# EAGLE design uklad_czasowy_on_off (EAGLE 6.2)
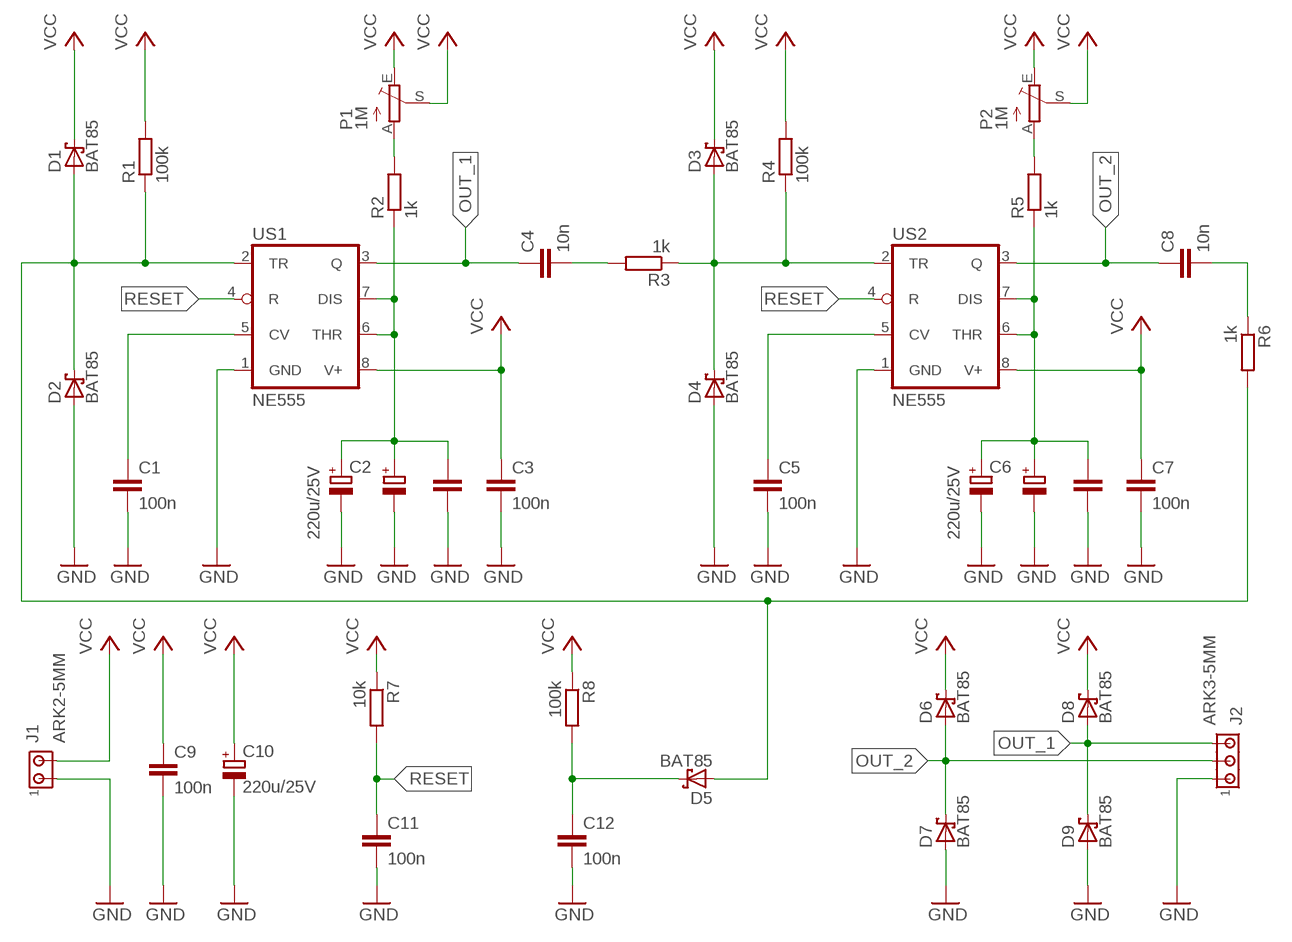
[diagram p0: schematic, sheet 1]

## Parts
C1  100n  C-EU050-025X075  [C050-025X075]
C2  220u/25V  CPOL-EUE3.5-10  [E3,5-10]
C2A  CPOL-EUE2.5-7  [E2,5-7]
C2B  C-EU050-025X075  [C050-025X075]
C3  100n  C-EU050-025X075  [C050-025X075]
C4  10n  C-EU050-025X075  [C050-025X075]
C5  100n  C-EU050-025X075  [C050-025X075]
C6  220u/25V  CPOL-EUE3.5-10  [E3,5-10]
C6A  CPOL-EUE2.5-7  [E2,5-7]
C6B  C-EU050-025X075  [C050-025X075]
C7  100n  C-EU050-025X075  [C050-025X075]
C8  10n  C-EU050-025X075  [C050-025X075]
C9  100n  C-EU050-025X075  [C050-025X075]
C10  220u/25V  CPOL-EUE2.5-6  [E2,5-6]
C11  100n  C-EU050-025X075  [C050-025X075]
C12  100n  C-EU050-025X075  [C050-025X075]
D1  BAT85  SCHOTTKY-DIODEDO35-7  [DO35-7]
D2  BAT85  SCHOTTKY-DIODEDO35-7  [DO35-7]
D3  BAT85  SCHOTTKY-DIODEDO35-7  [DO35-7]
D4  BAT85  SCHOTTKY-DIODEDO35-7  [DO35-7]
D5  BAT85  SCHOTTKY-DIODEDO35-7  [DO35-7]
D6  BAT85  SCHOTTKY-DIODEDO35-7  [DO35-7]
D7  BAT85  SCHOTTKY-DIODEDO35-7  [DO35-7]
D8  BAT85  SCHOTTKY-DIODEDO35-7  [DO35-7]
D9  BAT85  SCHOTTKY-DIODEDO35-7  [DO35-7]
J1  ARK2-5MM  [2PIN-5MM]
J2  ARK3-5MM  [3PIN-5MM]
P1  1M  TRIM_EU-B90P  [SP19L]
P2  1M  TRIM_EU-B90P  [SP19L]
R1  100k  R-EU_0207/7  [0207/7]
R2  1k  R-EU_0207/7  [0207/7]
R3  1k  R-EU_0207/7  [0207/7]
R4  100k  R-EU_0207/7  [0207/7]
R5  1k  R-EU_0207/7  [0207/7]
R6  1k  R-EU_0207/7  [0207/7]
R7  10k  R-EU_0207/7  [0207/7]
R8  100k  R-EU_0207/7  [0207/7]
US1  NE555  LM555N  [DIL08]
US2  NE555  LM555N  [DIL08]

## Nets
GND: C1.2 C2.- C2A.- C2B.2 C3.2 C5.2 C6.- C6A.- C6B.2 C7.2 C9.2 C10.- C11.2 C12.2 D2.A D4.A D7.A D9.A J1.P$1 J2.P$1 US1.1(GND) US2.1(GND)
N$1: C2.+ C2A.+ C2B.1 R2.1 US1.6(THR) US1.7(DIS)
N$2: P1.A R2.2
N$3: C1.1 US1.5(CV)
N$4: D1.A D2.C D5.A R1.1 R6.2 US1.2(TR)
N$5: C6.+ C6A.+ C6B.1 R5.1 US2.6(THR) US2.7(DIS)
N$6: P2.A R5.2
N$7: C5.1 US2.5(CV)
N$8: D3.A D4.C R3.1 R4.1 US2.2(TR)
N$9: C4.2 R3.2
N$10: C8.2 R6.1
N$11: C12.1 D5.C R8.2
OUT_1: C4.1 D8.A D9.C J2.P$3 US1.3(Q)
OUT_2: C8.1 D6.A D7.C J2.P$2 US2.3(Q)
RESET: C11.1 R7.2 US1.4(R) US2.4(R)
VCC: C3.1 C7.1 C9.1 C10.+ D1.C D3.C D6.C D8.C J1.P$2 P1.E P1.S P2.E P2.S R1.2 R4.2 R7.1 R8.1 US1.8(V+) US2.8(V+)

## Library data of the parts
C1 C2B C3-C5 C6B C7-C9 C11 C12 = rcl:C-EU: CAPACITOR, European symbol
C2 C2A C6 C6A C10 = rcl:CPOL-EU: POLARIZED CAPACITOR, European symbol
D1-D9 = diode:SCHOTTKY-DIODE: Schottky Diode
J1 = zlacza_futrzak:ARK2: ARK 2
J2 = zlacza_futrzak:ARK3: ARK 3 Raster 5mm i 3,5mm
P1 P2 = pot:TRIM_EU-: POTENTIOMETER
R1-R8 = rcl:R-EU_: RESISTOR, European symbol
US1 US2 = linear:*555: TIMER

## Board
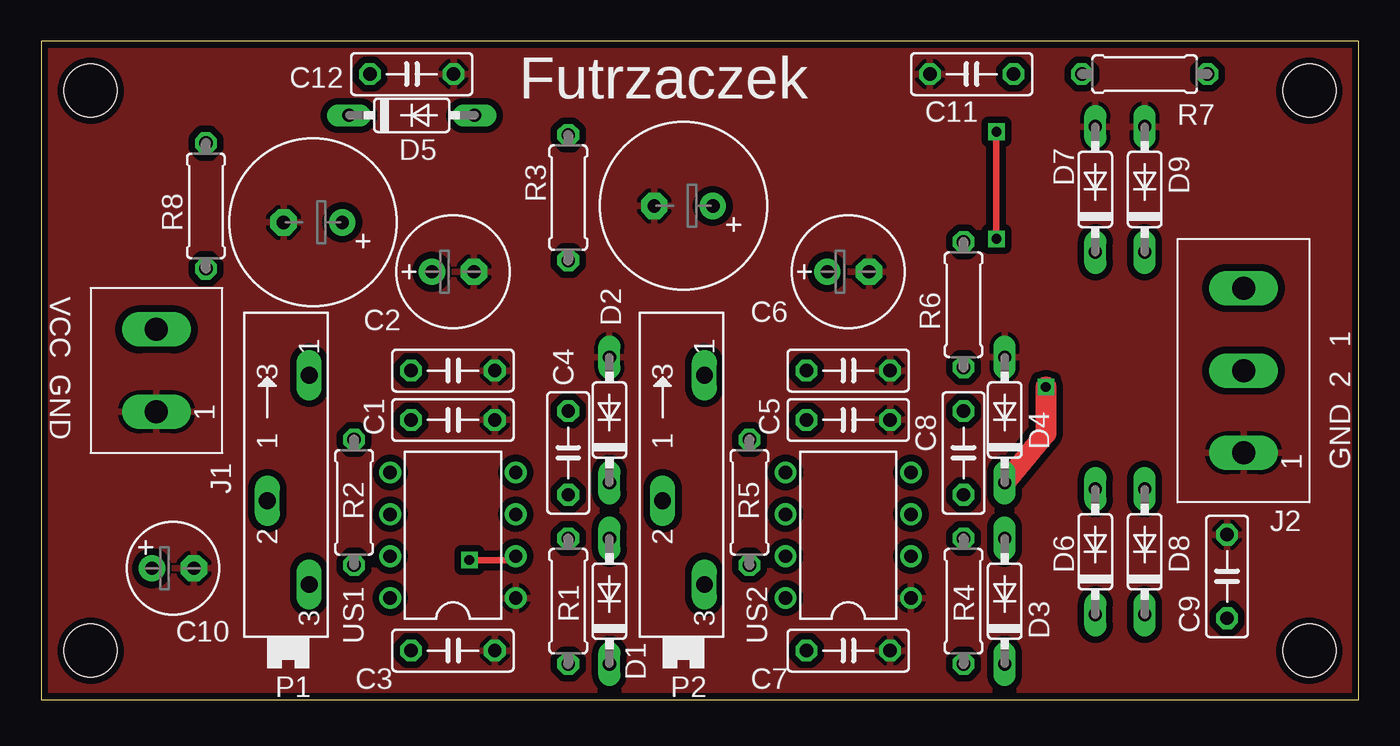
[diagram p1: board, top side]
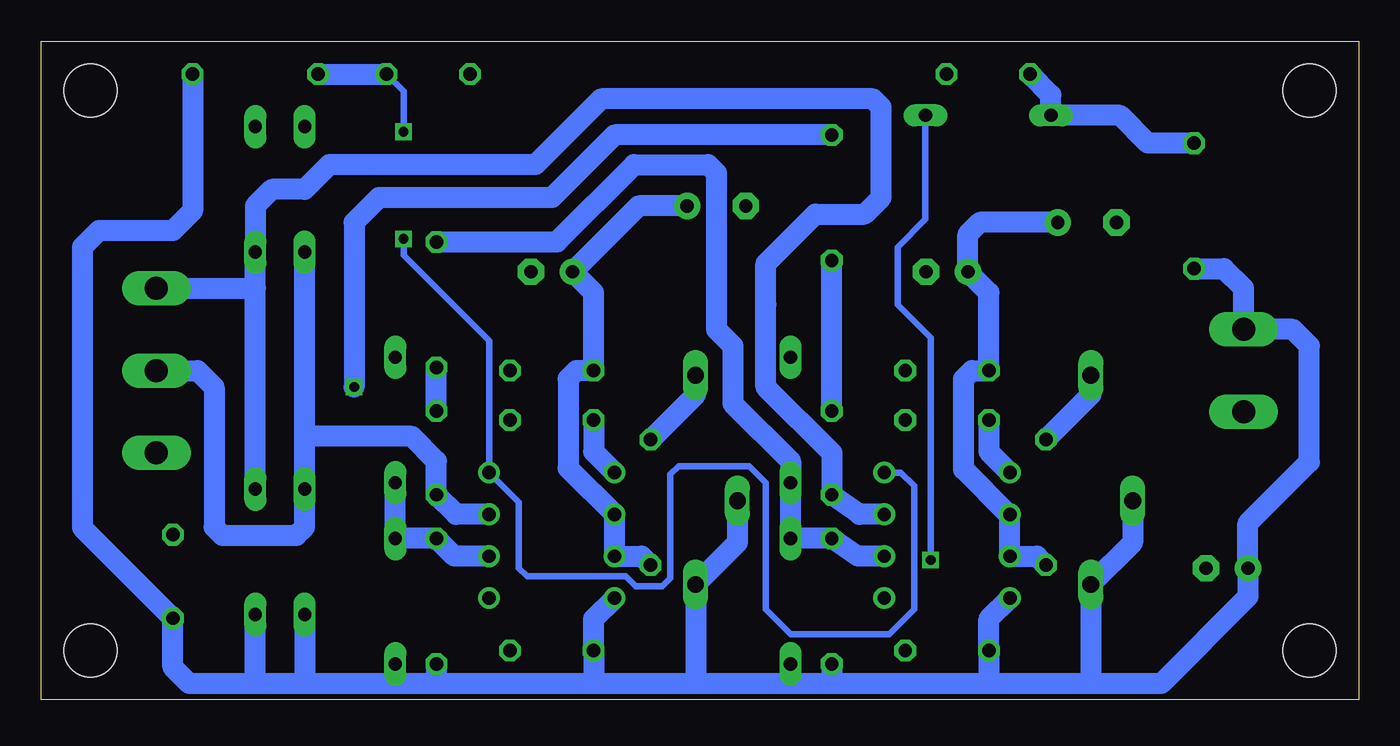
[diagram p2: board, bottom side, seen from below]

Size 80 x 40 mm. Coordinates in mm from the lower left corner, seen from the top.
Outline: 0,0 80,0 80,40 0,40 0,0
Copper layers (1*16): Top 0.035mm / dielectric 1.5mm / Bottom 0.035mm
Design rules: minimum track width 10mil, minimum drill 23mil, track to track 8mil, track to pad 8mil, pad to pad 8mil, via to via 8mil, smd to smd 8mil, copper to edge 10mil, drill to drill 8mil, minimum pad ring 10mil, minimum via ring 8mil, stop-mask expansion 4mil, vias tented up to drill 0mil, thermal gap 10mil
Holes 3.2 mm at 3,3 3,37 77,37 77,3

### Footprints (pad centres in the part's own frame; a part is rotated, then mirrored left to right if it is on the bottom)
C050-025X075 = drill 0.813 octagon: 1 -2.54,0; 2 2.54,0
E3,5-10 = drill 0.813 pad 1.6: + -1.778,0 | drill 0.813 pad 1.6 octagon: - 1.778,0
E2,5-7 = drill 0.813 pad 1.6: + -1.27,0 | drill 0.813 pad 1.6 octagon: - 1.27,0
E2,5-6 = drill 0.813 pad 1.6: + -1.27,0 | drill 0.813 pad 1.6 octagon: - 1.27,0
DO35-7 = drill 0.813 long: A 3.81,0; C -3.81,0
2PIN-5MM = drill 1.4 long: P$1 -2.5,0; P$2 2.5,0
3PIN-5MM = drill 1.4 long: P$1 -5,0; P$2 0,0; P$3 5,0
SP19L = drill 1.016 long: A 5.715,-1.27; E -6.985,-1.27; S -1.905,1.27
0207/7 = drill 0.813 octagon: 1 -3.81,0; 2 3.81,0
DIL08 = drill 0.813 pad 1.27: 1 -3.81,-3.81; 2 -1.27,-3.81; 3 1.27,-3.81; 4 3.81,-3.81; 5 3.81,3.81; 6 1.27,3.81; 7 -1.27,3.81; 8 -3.81,3.81

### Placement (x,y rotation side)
C1  25,17 0 top
C2  16.5,29 180 top
C2A  25,26 0 top
C2B  25,20 0 top
C3  25,3 0 top
C4  32,15 90 top
C5  49,17 0 top
C6  39,30 180 top
C6A  49,26 0 top
C6B  49,20 0 top
C7  49,3 0 top
C8  56,15 90 top
C9  72,7.5 90 top
C10  8,8 0 top
C11  56.5,38 180 top
C12  22.5,38 0 top
D1  34.5,6 90 top
D2  34.5,17 90 top
D3  58.5,6 90 top
D4  58.5,17 90 top
D5  22.5,35.5 0 top
D6  64,9 90 top
D7  64,31 90 top
D8  67,9 90 top
D9  67,31 90 top
J1  7,20 90 top
J2  73,20 90 top
P1  15,14 90 top
P2  39,14 90 top
R1  32,6 270 top
R2  19,12 90 top
R3  32,30.5 270 top
R4  56,6 270 top
R5  43,12 90 top
R6  56,24 90 top
R7  67,38 180 top
R8  10,30 90 top
US1  25,10 90 top
US2  49,10 90 top

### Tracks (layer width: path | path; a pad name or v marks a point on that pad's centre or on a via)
GND
  pour Top (isolate 0.406): 0,40 80,40 80,0 0,0
N$1
  Bottom 1.27: R2.1 19.54,8.73 US1.7 US1.6 21.27,11.27 24,14 24,19.5 23.5,20 C2B.1 22.46,24.73 C2A.+ 23.73,28.27 23,29 C2.+
N$2
  Bottom 1.27: P1.A 16.27,18.54 R2.2
N$3
  Bottom 1.27: C1.1 22.46,15.08 US1.5
N$4  (via drill 0.6)
  Top 0.406: v26,8.5 28.58,8.5 US1.2
  Bottom 0.406: D5.A 26.31,29.19 28,27.5 28,24 26,22 v26,8.5
  Bottom 1.27: US1.2 30.42,8.73 R1.1 D1.A D2.C 34.5,14.5 38,18 38,21.5 39,22.5 39,32 39.5,32.5 44,32.5 48.69,27.81 R6.2
N$5
  Bottom 1.27: R5.1 43.54,8.73 US2.7 US2.6 48,14.08 48,19.5 47.5,20 C6B.1 46.46,24.73 C6A.+ 43.73,30 C6.+
N$6
  Bottom 1.27: P2.A 40.27,18.54 R5.2
N$7
  Bottom 1.27: C5.1 46.46,15.08 US2.5
N$8  (via drill 0.6)
  Top 1.27: v61,19 61,16.19 D4.C
  Bottom 1.27: US2.2 54.92,8.73 R4.1 D3.A D4.C | R3.1 45.19,34.31 49,30.5 59.5,30.5 61,29 v61,19
N$9
  Bottom 1.27: C4.2 R3.2
N$10
  Bottom 1.27: C8.2 R6.1
N$11
  Bottom 1.27: R8.2 12.81,33.81 14.5,35.5 D5.C 18.69,36.73 C12.1
OUT_1
  Bottom 1.27: US1.3 30.31,11.27 C4.1 32,15 36,19 36,24 36,26.5 33,29.5 30,29.5 29,30.5 29,36 29.5,36.5 46,36.5 50,32.5 62.5,32.5 64,31 66,31 67,30 D9.C 67,25 | D8.A 67,25 | J2.P$3 67,25
OUT_2
  Bottom 1.27: US2.3 54.81,11.27 C8.1 56,14.5 57.5,16 64,16 | 64,16 D6.A 64,10.5 64.5,10 69,10 69.5,10.5 69.5,19 70.5,20 J2.P$2 | 64,16 D7.C
RESET  (via drill 0.6)
  Top 0.406: v58,28 v58,34.5
  Bottom 0.406: US1.4 27.81,13.81 27,13 27,5.5 28.5,4 34.5,4 36,5.5 36,13.2 37,14.2 41.3,14.2 41.8,13.7 41.8,7.4 42.3,6.9 43.9,6.9 44.5,7.5 50.5,7.5 51,8 51,12 US2.4 52.81,21.81 58,27 v58,28 | v58,34.5 58,36.96 C11.1
  Bottom 1.27: R7.2 C11.1
VCC
  Bottom 1.27: 16,1 12,1 6.73,6.27 C10.+ 6.73,10.73 3,14.46 3,21.5 4,22.5 J1.P$2 7,25 8.19,26.19 R8.1 | 16,1 22.5,1 | 22.5,1 32,1 | 32,1 34.5,1 | 34.5,1 40,1 | 40,1 46.5,1 | 46.5,1 56,1 | 56,1 58.5,1 | 58.5,1 64,1 | 64,1 67,1 | 67,1 D8.C | D6.C 64,1 | D3.C 58.5,1 | R4.2 56,1 | 46.5,1 46.46,1.04 C7.1 46.46,4.92 US2.8 | 40,1 40.27,1.27 P2.E 37.73,9.55 P2.S | P1.S 13.73,9.55 P1.E 16.27,1.27 16,1 | 22.5,1 22.46,1.04 C3.1 22.46,4.92 US1.8 | D1.C 34.5,1 | R1.2 32,1 | 67,1 71,1 72,2 C9.1 77.5,10.46 77.5,27.5 76.5,28.5 72,28.5 70.81,29.69 R7.1

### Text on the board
tPlace: Futrzaczek | VCC GND | GND 2 1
